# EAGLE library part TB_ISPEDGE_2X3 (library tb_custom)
AVR-ISP connector an Platinenrand
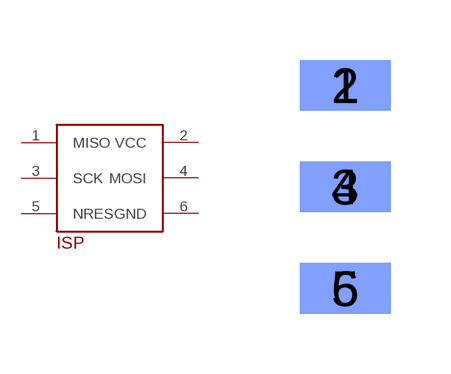
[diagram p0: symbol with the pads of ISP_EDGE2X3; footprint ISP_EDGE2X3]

Designator prefix -

## TB_ISPEDGE_2X3  [ISP_EDGE2X3]
1  MISO
2  VCC
3  SCK
4  MOSI
5  NRES
6  GND

## Footprint ISP_EDGE2X3 (pad centres in mm)
smd 2.286 x 1.27: 1 -0.127,2.54; 3 -0.127,0; 5 -0.127,-2.54
smd 2.286 x 1.27 bottom: 2 -0.127,2.54; 4 -0.127,0; 6 -0.127,-2.54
